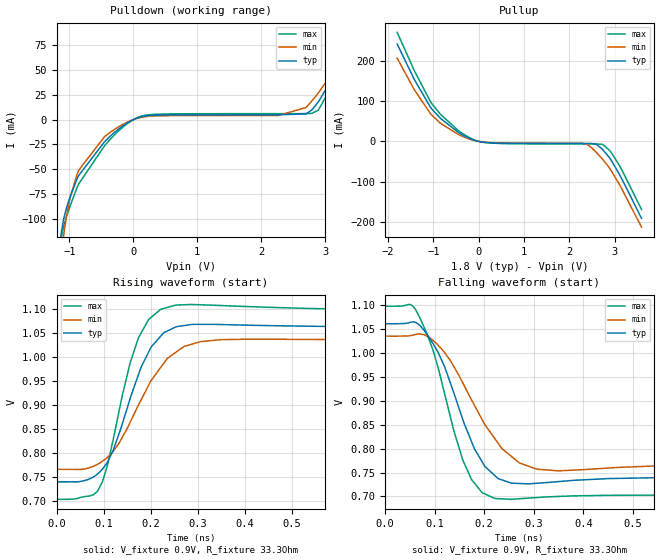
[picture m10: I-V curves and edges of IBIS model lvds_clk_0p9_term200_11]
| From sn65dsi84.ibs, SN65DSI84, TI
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|   Model
[Model]   lvds_clk_0p9_term200_11
Model_type   Output
Polarity   Non-Inverting
Vmeas = 0.9
Vref = 0.9
Cref = 1pF
Rref = 50
|   typ   min   max
C_comp   0.4797pF   0.3035pF   0.7186pF
[Voltage Range]   1.8   1.65   1.95
[Temperature Range]   27   125   -40
[Pullup Reference]   1.8   1.65   1.95
[Pulldown Reference]   -0   -0   -0
[Power Clamp Reference]   1.8   1.65   1.95
[GND Clamp Reference]   -0   -0   -0
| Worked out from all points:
|   slope of the pulldown table from 0 to 0.27 V, typ, clamps not added: 63.6 ohm
|   slope of the pullup table from 0 to 0.27 V, typ, clamps not added: 76.3 ohm
|   falling waveform, V_fixture 0.9V, R_fixture 33.3Ohm: 20-80 % time 69.6ps typ, 89.1ps min, 62.9ps max; typ from 1.06 V to 0.739 V
|   rising waveform, V_fixture 0.9V, R_fixture 33.3Ohm: 20-80 % time 69.3ps typ, 91.5ps min, 56.8ps max; typ from 0.739 V to 1.06 V
[Pulldown]
|   Voltage   I(typ)   I(min)   I(max)
-1.8V     -662.8mA   -697.9mA   -653.3mA
-1.141V   -120.2mA   -145.2mA   -123.4mA
-1.087V   -100mA     -116mA     -107.2mA
-990mV    -78.04mA   -79.29mA   -87.37mA
-855mV    -56.34mA   -51.07mA   -64.87mA
-450mV    -22.28mA   -17.17mA   -26.37mA
-190.8mV  -7.548mA   -5.75mA    -9.039mA
79.2mV    2.068mA    1.611mA    2.505mA
2.261V    4.9mA      4.126mA    6.05mA
2.698V    5.78mA     12.21mA    6.095mA
2.893V    18.06mA    27.07mA    9.681mA
3.595V    93.26mA    90.74mA    91.15mA
[Pullup]
|   Voltage   I(typ)   I(min)   I(max)
-1.8V     242.5mA    207.5mA    271.8mA
-1.417V   153.4mA    127.9mA    175.1mA
-1.049V   82.63mA    67.15mA    96.24mA
-450mV    22.49mA    17.22mA    27.03mA
-126mV    4.234mA    3.233mA    5.131mA
154.8mV   -2.654mA   -2.236mA   -3.082mA
2.374V    -5.255mA   -6.299mA   -6.399mA
2.601V    -7.407mA   -27.98mA   -6.525mA
2.741V    -21.24mA   -45.38mA   -8.028mA
2.903V    -43.39mA   -69.1mA    -24.76mA
3.136V    -88.4mA    -113.6mA   -66.04mA
3.595V    -191.9mA   -213.8mA   -169.6mA
[Ramp]
R_load = 33.3
|   typ   min   max
dV/dt_r   0.193374/6.93398e-11   0.162176/9.14751e-11   0.236776/5.67874e-11
dV/dt_f   0.192998/6.95686e-11   0.161794/8.91115e-11   0.236831/6.29362e-11
[Falling Waveform]
V_fixture = 0.9V
V_fixture_min = 0.9V
V_fixture_max = 0.9V
R_fixture = 33.3Ohm
C_fixture = 0F
|   Time   V(typ)   V(min)   V(max)
0s        1.061V     1.035V     1.098V
50ps      1.063V     1.036V     1.101V
63.2ps    1.063V     1.039V     1.088V
107.7ps   999.9mV    1.015V     966.8mV
156.8ps   860.9mV    937.4mV    776.4mV
195.7ps   772.7mV    860.8mV    708.1mV
221.6ps   743.6mV    820.7mV    695.8mV
270.8ps   727.2mV    770.2mV    695.3mV
349.2ps   731.1mV    753.6mV    700.1mV
1ns       739.3mV    765.4mV    702.8mV
[Rising Waveform]
V_fixture = 0.9V
V_fixture_min = 0.9V
V_fixture_max = 0.9V
R_fixture = 33.3Ohm
C_fixture = 0F
|   Time   V(typ)   V(min)   V(max)
0s        739.3mV    765.4mV    702.8mV
87.21ps   755.7mV    776mV      719.8mV
108.1ps   780.3mV    790.6mV    773.4mV
120.9ps   806.1mV    803.8mV    829.7mV
156.8ps   914.2mV    864.4mV    989.1mV
174.3ps   963.4mV    899.8mV    1.041V
221.6ps   1.044V     978.4mV    1.1V
270.8ps   1.066V     1.022V     1.109V
349.2ps   1.068V     1.036V     1.108V
1ns       1.062V     1.036V     1.097V
